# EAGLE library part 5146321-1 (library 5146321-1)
Body Features: Connector Profile Standard | Primary Product Color Black | Configuration Features: PCB Mount Orientation Right Angle | Number of Positions 68 | Number of Card Slots 1 | Number of Rows 5 | Contact Features: Contact Type Pin | Contact Current Rating (Max) .1 AMP | Contact Base Material Brass | Contact Underplating Material Nickel | Contact Mating Area Plating Material Thickness 30 MICIN | Contact Layout Staggered | Contact Mating Area Plating Material Gold | PCB Contact Termination Area Plating Source: Datasheet
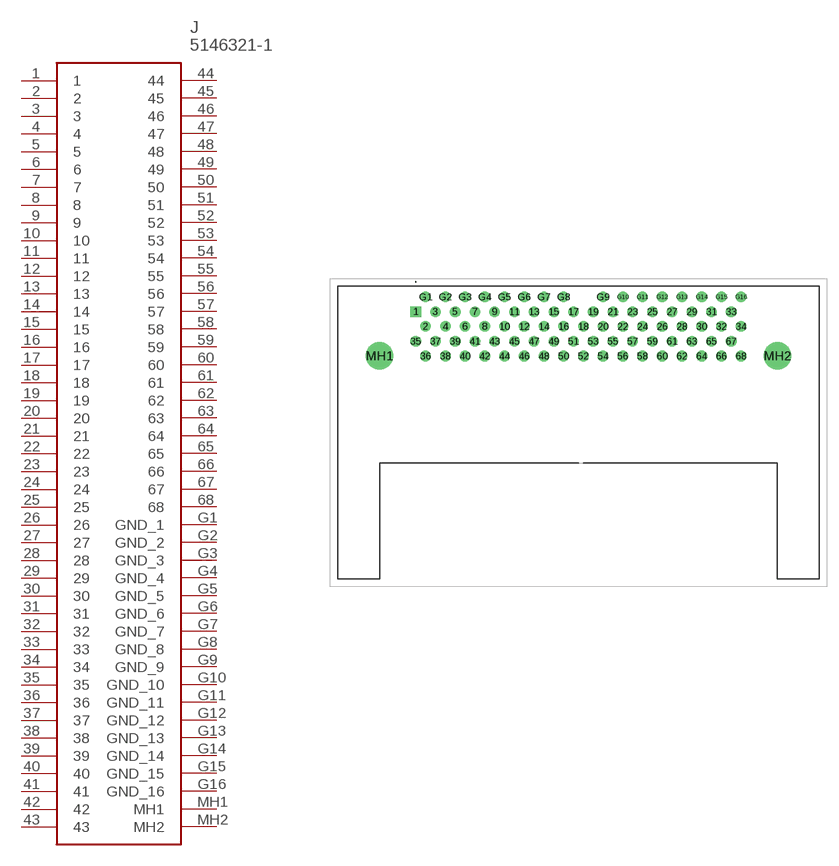
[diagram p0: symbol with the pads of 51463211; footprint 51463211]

Designator prefix J

## 5146321-1 (Description: Body Features: Connector Profile Standard | Primary Product Color Black | Configuration Features: PCB Mount Orientation Right Angle | Number of Positions 68 | Number of Card Slots 1 | Number of Rows 5 | Contact Features: Contact Type Pin | Contact Current Rating (Max) .1 AMP | Contact Base Material Brass | Contact Underplating Material Nickel | Contact Mating Area Plating Material Thickness 30 MICIN | Contact Layout Staggered | Contact Mating Area Plating Material Gold | PCB Contact Termination Area Plating; Height: 7.32mm; Manufacturer_Name: TE Connectivity; Manufacturer_Part_Number: 5146321-1; Mouser_Part_Number: 571-5146321-1; Mouser_Price-Stock: https://www.mouser.co.uk/ProductDetail/TE-Connectivity-AMP/5146321-1?qs=bwpFY26eRVc85mTfU6Ed9w%3D%3D)  [51463211]
1  1
2  2
3  3
4  4
5  5
6  6
7  7
8  8
9  9
10  10
11  11
12  12
13  13
14  14
15  15
16  16
17  17
18  18
19  19
20  20
21  21
22  22
23  23
24  24
25  25
26  26
27  27
28  28
29  29
30  30
31  31
32  32
33  33
34  34
35  35
36  36
37  37
38  38
39  39
40  40
41  41
42  42
43  43
44  44
45  45
46  46
47  47
48  48
49  49
50  50
51  51
52  52
53  53
54  54
55  55
56  56
57  57
58  58
59  59
60  60
61  61
62  62
63  63
64  64
65  65
66  66
67  67
68  68
G1  GND_1
G2  GND_2
G3  GND_3
G4  GND_4
G5  GND_5
G6  GND_6
G7  GND_7
G8  GND_8
G9  GND_9
G10  GND_10
G11  GND_11
G12  GND_12
G13  GND_13
G14  GND_14
G15  GND_15
G16  GND_16
MH1  MH1
MH2  MH2

## Footprint 51463211 (pad centres in mm)
5146321-1-1
drill 0.84 pad 1.365 square: 1 0,0
drill 0.84 pad 1.365: 2 1.27,-1.905; 3 2.54,0; 4 3.81,-1.905; 5 5.08,0; 6 6.35,-1.905; 7 7.62,0; 8 8.89,-1.905; 9 10.16,0; 10 11.43,-1.905; 11 12.7,0; 12 13.97,-1.905; 13 15.24,0; 14 16.51,-1.905; 15 17.78,0; 16 19.05,-1.905; 17 20.32,0; 18 21.59,-1.905; 19 22.86,0; 20 24.13,-1.905; 21 25.4,0; 22 26.67,-1.905; 23 27.94,0; 24 29.21,-1.905; 25 30.48,0; 26 31.75,-1.905; 27 33.02,0; 28 34.29,-1.905; 29 35.56,0; 30 36.83,-1.905; 31 38.1,0; 32 39.37,-1.905; 33 40.64,0; 34 41.91,-1.905; 35 0,-3.81; 36 1.27,-5.715; 37 2.54,-3.81; 38 3.81,-5.715; 39 5.08,-3.81; 40 6.35,-5.715; 41 7.62,-3.81; 42 8.89,-5.715; 43 10.16,-3.81; 44 11.43,-5.715; 45 12.7,-3.81; 46 13.97,-5.715; 47 15.24,-3.81; 48 16.51,-5.715; 49 17.78,-3.81; 50 19.05,-5.715; 51 20.32,-3.81; 52 21.59,-5.715; 53 22.86,-3.81; 54 24.13,-5.715; 55 25.4,-3.81; 56 26.67,-5.715; 57 27.94,-3.81; 58 29.21,-5.715; 59 30.48,-3.81; 60 31.75,-5.715; 61 33.02,-3.81; 62 34.29,-5.715; 63 35.56,-3.81; 64 36.83,-5.715; 65 38.1,-3.81; 66 39.37,-5.715; 67 40.64,-3.81; 68 41.91,-5.715; G1 1.27,1.905; G2 3.81,1.905; G3 6.35,1.905; G4 8.89,1.905; G5 11.43,1.905; G6 13.97,1.905; G7 16.51,1.905; G8 19.05,1.905; G9 24.13,1.905; G10 26.67,1.905; G11 29.21,1.905; G12 31.75,1.905; G13 34.29,1.905; G14 36.83,1.905; G15 39.37,1.905; G16 41.91,1.905
drill 2.36 pad 3.54: MH1 -4.67,-5.715; MH2 46.59,-5.715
